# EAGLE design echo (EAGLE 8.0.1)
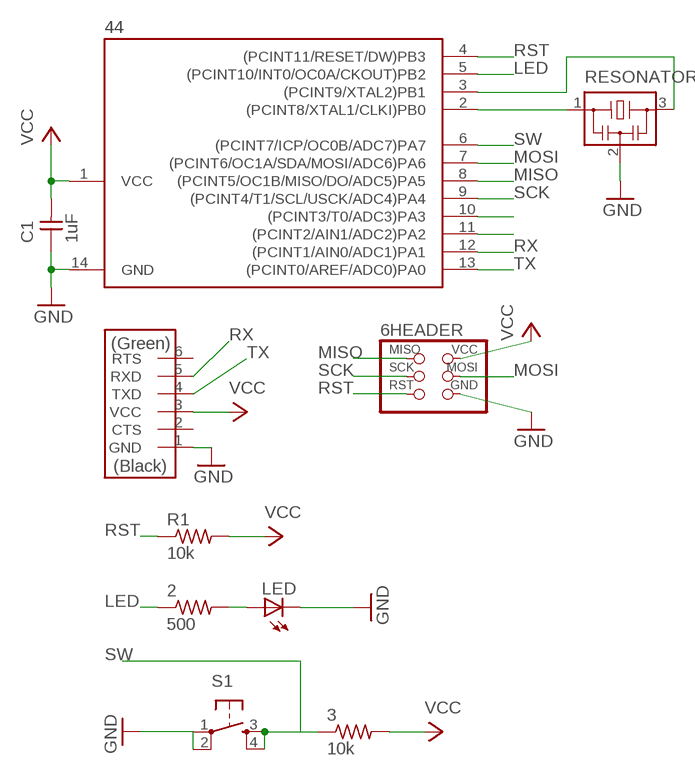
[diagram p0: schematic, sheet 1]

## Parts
2  500  RES-US1206FAB  [R1206FAB]
3  10k  RES-US1206FAB  [R1206FAB]
6HEADER  AVRISPSMD  [2X03SMD]
44  ATTINY44-SSU  [SOIC14]
C1  1uF  CAP-UNPOLARIZEDFAB  [C1206FAB]
LED  LEDFAB1206  [LED1206FAB]
R1  10k  RES-US1206FAB  [R1206FAB]
RESONATOR  RESONATOR  [EFOBM]
S1  6MM_SWITCH6MM_SWITCH  [6MM_SWITCH]
U$4  con  FTDI-SMD-HEADER  [1X06SMD]

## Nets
GND: 6HEADER.6(GND) 44.14(GND) C1.1 LED.2(C) RESONATOR.2 S1.1(P) S1.2(P1) U$4.1(GND)
LED: 2.1 44.5((PCINT10/INT0/OC0A/CKOUT)PB2)
MISO: 6HEADER.1(MISO) 44.8((PCINT5/OC1B/MISO/DO/ADC5)PA5)
MOSI: 6HEADER.4(MOSI) 44.7((PCINT6/OC1A/SDA/MOSI/ADC6)PA6)
N$1: 44.2((PCINT8/XTAL1/CLKI)PB0) RESONATOR.1
N$2: 44.3((PCINT9/XTAL2)PB1) RESONATOR.3
N$3: 2.2 LED.1(A)
N$7: 44.10((PCINT3/T0/ADC3)PA3)
N$8: 44.11((PCINT2/AIN1/ADC2)PA2)
RST: 6HEADER.5(RST) 44.4((PCINT11/RESET/DW)PB3) R1.1
RX: 44.12((PCINT1/AIN0/ADC1)PA1) U$4.5(RXD)
SCK: 6HEADER.3(SCK) 44.9((PCINT4/T1/SCL/USCK/ADC4)PA4)
SW: 3.1 44.6((PCINT7/ICP/OC0B/ADC7)PA7) S1.3(S) S1.4(S1)
TX: 44.13((PCINT0/AREF/ADC0)PA0) U$4.4(TXD)
VCC: 3.2 6HEADER.2(VCC) 44.1(VCC) C1.2 R1.2 U$4.3(VCC)
Unconnected: U$4.2(CTS) U$4.6(RTS)

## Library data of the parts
2 3 R1 = fab:RES-US: Resistor (US Symbol)
6HEADER = fab:AVRISP
44 = fab:ATTINY44
C1 = fab:CAP-UNPOLARIZED
LED = fab:LED: LED
RESONATOR = fab:RESONATOR
S1 = fab:6MM_SWITCH: OMRON SWITCH
U$4 = fab:FTDI-SMD-HEADER

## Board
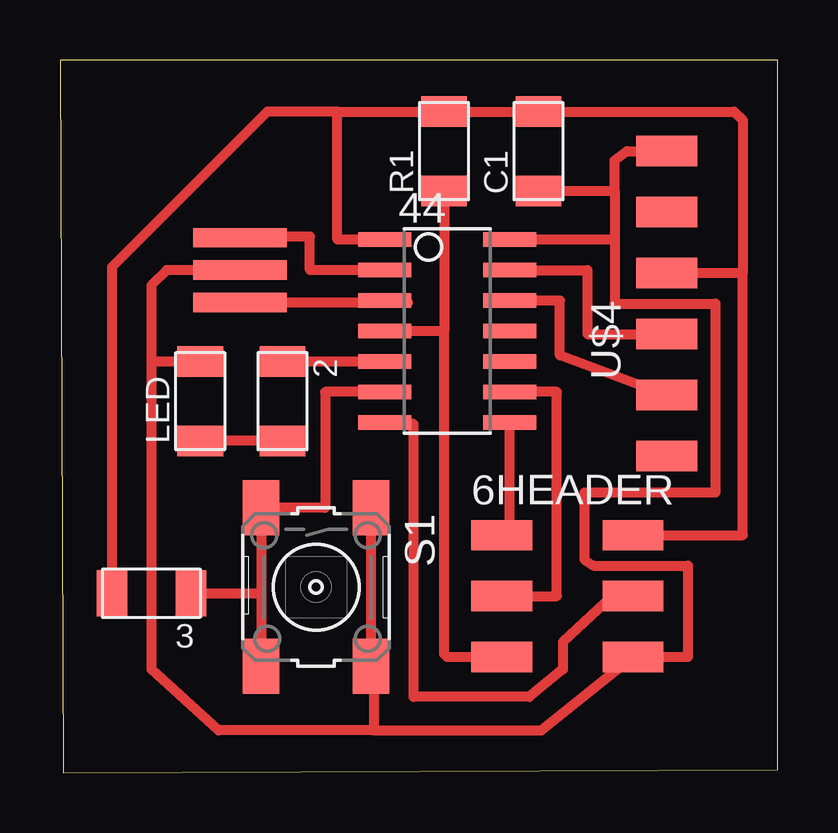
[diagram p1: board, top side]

Size 29.9 x 29.71 mm. Coordinates in mm from the lower left corner, seen from the top.
Outline: 0.13,0 29.9,0.13 29.9,29.71 0,29.71 0.13,0
Copper layers (1*16): Top 0.035mm / dielectric 1.5mm / Bottom 0.035mm
Design rules "default *": minimum track width 10mil, minimum drill 24mil, track to track 16mil, track to pad 16mil, pad to pad 16mil, via to via 16mil, smd to smd 16mil, copper to edge 40mil, drill to drill 8mil, minimum pad ring 10mil, minimum via ring 8mil, stop-mask expansion 4mil, vias tented up to drill 0mil, thermal gap 10mil

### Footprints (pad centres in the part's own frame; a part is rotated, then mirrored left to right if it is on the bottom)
R1206FAB = smd 1.27 x 1.905: 1 -1.651,0; 2 1.651,0
2X03SMD = smd 2.54 x 1.27: 1 -2.54,2.54; 2 2.92,2.54; 3 -2.54,0; 4 2.92,0; 5 -2.54,-2.54; 6 2.92,-2.54
SOIC14 = smd 0.61 x 2.21: 1 -3.81,-2.603; 2 -2.54,-2.603; 3 -1.27,-2.603; 4 0,-2.603; 5 1.27,-2.603; 6 2.54,-2.603; 7 3.81,-2.603; 8 3.81,2.603; 9 2.54,2.603; 10 1.27,2.603; 11 0,2.603; 12 -1.27,2.603; 13 -2.54,2.603; 14 -3.81,2.603
C1206FAB = smd 1.27 x 1.905: 1 -1.651,0; 2 1.651,0
LED1206FAB = smd 1.27 x 1.905: 1 -1.651,0; 2 1.651,0
EFOBM = smd 0.8 x 3.9: 1 -1.35,0; 2 0,0; 3 1.35,0
6MM_SWITCH = smd 2.286 x 1.524: 1 -3.302,2.286; 2 3.302,2.286; 3 -3.302,-2.286; 4 3.302,-2.286
1X06SMD = smd 2.54 x 1.27: 1 0,6.35; 2 0,3.81; 3 0,1.27; 4 0,-1.27; 5 0,-3.81; 6 0,-6.35

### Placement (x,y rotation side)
2  9.27,15.49 270 top
3  3.81,7.49 180 top
6HEADER  20.96,7.37 0 top
44  16.13,18.41 270 top
C1  19.94,25.91 90 top
LED  5.84,15.49 90 top
R1  16,25.91 90 top
RESONATOR  7.49,20.95 270 top
S1  10.67,7.75 270 top
U$4  25.27,19.56 0 top

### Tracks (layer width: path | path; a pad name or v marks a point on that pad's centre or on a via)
GND
  Top 0.406: 3.81,17.15 3.81,4.32 6.6,1.78 13.08,1.78 | 13.08,1.78 20.07,1.78 6HEADER.6 26.16,4.83 26.16,8.64 22.22,8.64 21.84,8.89 21.84,11.68 27.3,11.68 27.3,19.56 23.11,19.56 23.11,22.23 | 23.11,22.23 44.14 | LED.2 3.81,17.15 | RESONATOR.2 4.45,20.95 3.81,20.32 3.81,17.15 | C1.1 23.11,24.26 | 23.11,24.26 23.11,22.23 | 23.11,24.26 23.11,25.53 23.62,25.91 U$4.1 | S1.1 S1.2 13.08,4.45 13.08,1.78
LED
  Top 0.406: 44.5 2.1
MISO
  Top 0.406: 6HEADER.1 18.73,9.91 44.8
MOSI
  Top 0.406: 6HEADER.4 22.99,7.37 20.96,5.46 20.96,4.32 19.56,3.18 14.73,3.18 14.73,14.54 44.7
N$1
  Top 0.406: RESONATOR.1 7.54,22.35 10.41,22.35 10.41,20.95 44.2
N$2
  Top 0.406: RESONATOR.3 14.49,19.6 44.3
N$3
  Top 0.406: 2.2 LED.1
RST
  Top 0.406: 6HEADER.5 16.13,4.83 16,4.95 16,18.41 | 16,18.41 44.4 | R1.1 16,18.41
RX
  Top 0.406: U$4.5 20.83,17.4 20.83,19.69 44.12
SCK
  Top 0.406: 6HEADER.3 20.7,7.37 20.7,15.88 44.9
SW
  Top 0.406: 8.38,7.49 S1.3 11.05,11.05 11.05,15.88 44.6 | 8.38,7.49 S1.4 | 3.1 8.38,7.49
TX
  Top 0.406: 44.13 21.97,20.95 21.97,18.29 U$4.4
VCC
  Top 0.406: 6HEADER.2 28.45,9.91 28.45,20.83 | 28.45,20.83 U$4.3 | 11.56,27.56 R1.2 C1.2 | 11.56,27.56 8.64,27.56 2.16,21.08 3.2 | C1.2 20.7,27.81 | 28.45,20.83 28.45,27.19 28.08,27.56 C1.2 | 44.1 11.56,22.23 11.56,27.56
